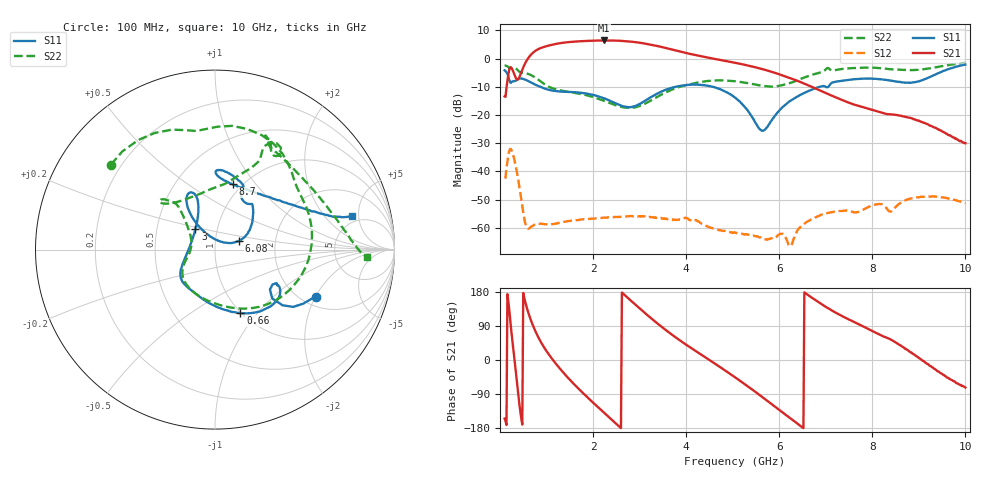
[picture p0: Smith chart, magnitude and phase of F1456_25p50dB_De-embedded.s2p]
! Integrated Device Technology
! Corporate Headquarters
! 6024 Silver Creek Valley Road
! San Jose, CA 95138  USA
! Phone:  1-408-284-8200
! Toll Free:  1-800-223-1366
! Webpage:  http://www.idt.com/
! Timing and RF Division
! 515 Groton Road, Suite 102
! Westford, MA 01886-6024
! Device:  F1456
! Description: 6-bit 0.5 dB Transmit Variable Gain Amplifier
! Frequency:  2100.0 -  2950.00 MHz
! Package:  6x6 mm Thin QFN Plastic Package: 28 pin
! State:  51
! Atten State:  25.5 dB
! Voltage:  +5.00 Volts
! Current:  216.952 mA
! Data:  The device was measured on a the F1455 evaluation board which has
!  individual transmission lines to the RF pins.  Data was collected
!  using a calibrated network analyzer.  The evaluation board was
!  de-embedded using a TRL calibration technique.
!  The reference plane is the edge of the package pin.
!  Pin  1 = CSb
!  Pin  2 = DATA
!  Pin  3 = CLK
!  Pin  4 = RSET
!  Pin  5 = GND
!  Pin  6 = RFIN  = Port 1
!  Pin  7 = GND
!  Pin  8 = NC
!  Pin  9 = NC
!  Pin 10 = NC
!  Pin 11 = NC
!  Pin 12 = NC
!  Pin 13 = NC
!  Pin 14 = /STBY
!  Pin 15 = GND
!  Pin 16 = RFOUT  = Port 2
!  Pin 17 = GND
!  Pin 18 = NC
!  Pin 19 = NC
!  Pin 20 = NC
!  Pin 21 = GND
!  Pin 22 = NC
!  Pin 23 = GND
!  Pin 24 = NC
!  Pin 25 = NC
!  Pin 26 = NC
!  Pin 27 = GND
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# GHz S dB R 50
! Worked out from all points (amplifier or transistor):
!   496 points, 100 MHz to 10 GHz, reference 50 ohm
!   highest |S21| = 6.5 dB at 2.24 GHz (marker M1)
!   |S21| within 3 dB of that: 832.8 MHz to 3.645 GHz (2.813 GHz wide, 126 % of centre)
!   unconditionally stable (mu >= 1): start of sweep to end of sweep
!   at 1.74 GHz: K = 154.62, MAG = 6.7 dB, |S12| = -57.1 dB
!   at 5.06 GHz: K = 588.91, MAG = -0.6 dB, |S12| = -61.8 dB
!   at 10 GHz: K = 628.26, MAG = -20.4 dB, |S12| = -51.2 dB
!   S11 on the Smith chart (normalised r, x): 100 MHz: 2.37, -2.03; 660 MHz: 0.99, -0.82; 3 GHz: 0.78, +0.18; 6.08 GHz: 1.30, +0.13; 8.7 GHz: 0.91, +0.77; 10 GHz: 4.20, +4.09
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0.1  -4.12 -24.9  -13.37 -154.7  -42.28 50.1  -2.52 140.8
0.24  -8.52 -31.1  -3.09 81.4  -32.20 -77.0  -3.44 94.6
0.32  -7.95 -29.4  -6.02 -6.7  -36.58 -155.0  -3.24 67.8
0.42  -7.02 -36.8  -6.43 -120.0  -45.69 140.5  -4.67 40.6
0.54  -7.40 -53.7  -1.69 155.1  -58.12 125.5  -5.12 16.7
0.66  -8.39 -68.2  1.30 106.7  -59.75 144.2  -5.76 -10.7
0.84  -9.82 -86.8  3.52 56.3  -58.60 117.3  -7.65 -48.5
1.16  -11.41 -113.4  5.09 -3.4  -58.63 82.1  -10.68 -94.6
1.42  -11.72 -127.7  5.79 -41.3  -57.77 64.7  -11.61 -119.1
1.76  -12.14 -140.7  6.21 -84.5  -57.05 46.6  -12.58 -139.6
2.24  -14.09 -156.0  6.46 -139.6  -56.42 26.9  -14.97 -158.4
2.6  -16.64 179.9  6.32 -179.8  -56.09 13.2  -17.08 -175.5
3  -16.06 134.1  5.65 136.2  -55.87 -5.6  -16.81 156.5
3.4  -12.23 112.2  4.42 94.8  -56.42 -22.1  -13.39 137.7
4.12  -9.21 113.1  1.56 30.7  -57.44 -55.7  -8.94 132.0
5.06  -13.92 125.4  -1.49 -46.5  -61.78 -102.0  -8.03 139.1
5.64  -25.61 69.2  -3.71 -98.0  -63.76 -152.9  -9.64 123.5
6.08  -17.07 19.9  -6.00 -139.2  -62.16 169.2  -9.33 92.0
6.7  -10.99 41.5  -9.99 164.5  -56.95 150.4  -5.77 65.2
8.36  -7.69 88.1  -19.70 56.4  -54.15 67.7  -3.71 62.3
8.7  -8.48 74.7  -20.62 30.0  -50.29 72.2  -4.01 51.1
10  -2.11 13.8  -29.98 -72.8  -51.21 -23.9  -1.46 -2.6
